FUNCTION "Interfaccia Destacker" : VOID
TITLE =Communication to previous cell
//
VERSION : 0.1

BEGIN
NETWORK
TITLE =Stops Out
//
//
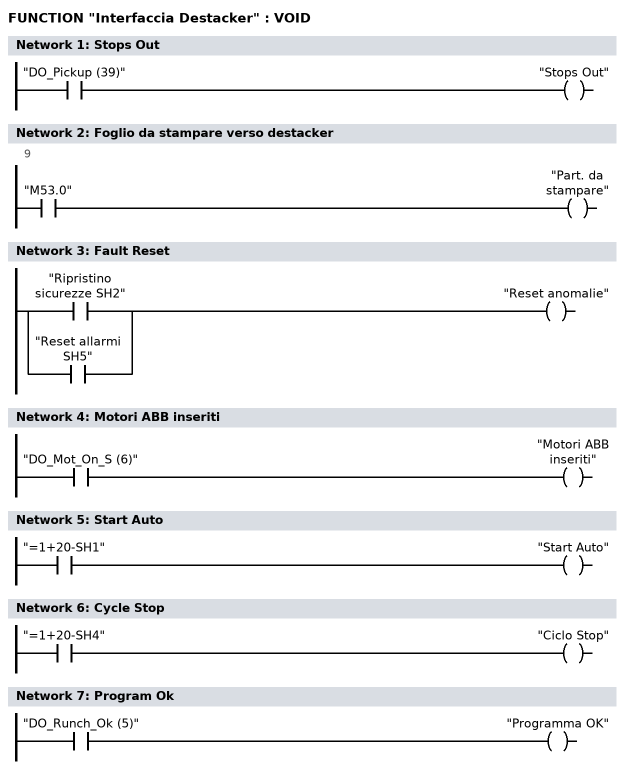
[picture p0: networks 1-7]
      U     "DO_Pickup (39)";
      =     "Stops Out";
NETWORK
TITLE =Foglio da stampare verso destacker
//9
      U     "M53.0";
      =     "Part. da stampare";
NETWORK
TITLE =Fault Reset

      O     "Ripristino sicurezze SH2";
      O     "Reset allarmi SH5";
      =     "Reset anomalie";
NETWORK
TITLE =Motori ABB inseriti

      U     "DO_Mot_On_S (6)";
      =     "Motori ABB inseriti";
NETWORK
TITLE =Start Auto

      U     "=1+20-SH1";
      =     "Start Auto";
NETWORK
TITLE =Cycle Stop

      U     "=1+20-SH4";
      =     "Ciclo Stop";
NETWORK
TITLE =Program Ok

      U     "DO_Runch_Ok (5)";
      =     "Programma OK";
NETWORK
TITLE =Cam Check Double Sheet Sensor

      U(    ;
      U     "vacuostato 1 ok";
      UN    "DO_Pickup (39)";
      L     S5T#1S;
      SE    T      2;
      NOP   0;
      NOP   0;
      NOP   0;
      U     T      2;
      )     ;
      U(    ;
      O     "DO_Motion (40)";
      O     "Selez.ciclo sing.ABB";
      )     ;
      =     "Cam contr. doppio foglio";
NETWORK
TITLE =Mode Selector Programming Mode
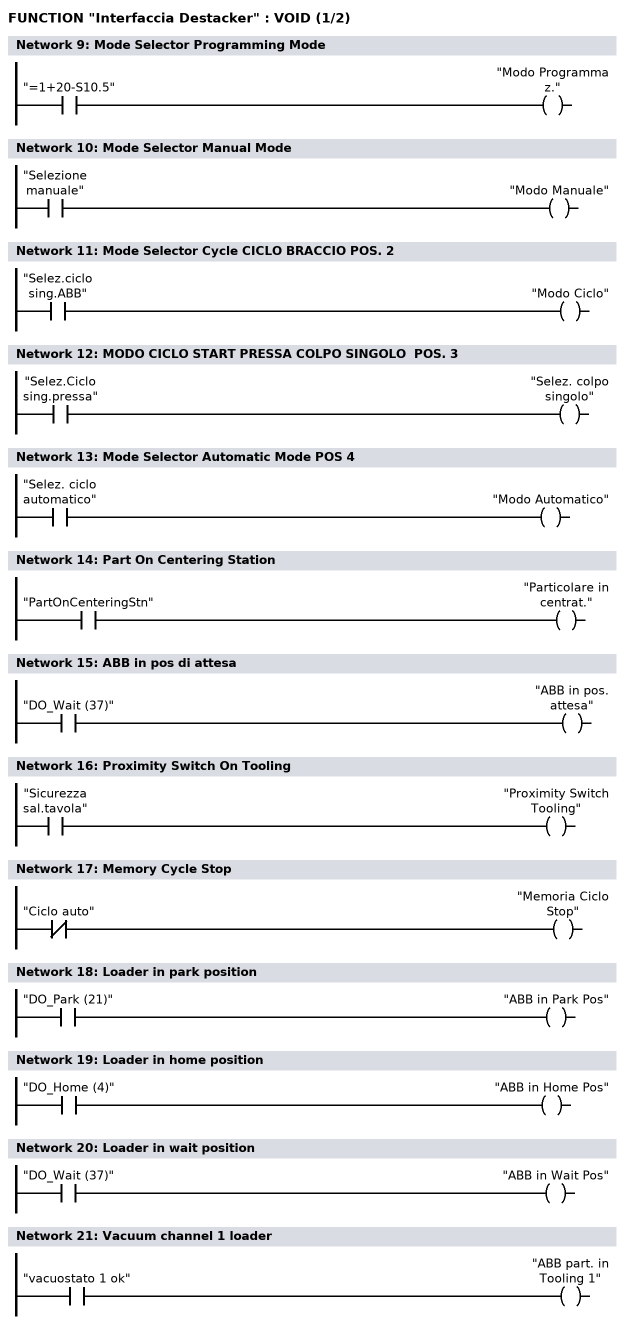
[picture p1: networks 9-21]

      U     "=1+20-S10.5";
      =     "Modo Programmaz.";
NETWORK
TITLE =Mode Selector Manual Mode

      U     "Selezione manuale";
      =     "Modo Manuale";
NETWORK
TITLE =Mode Selector Cycle CICLO BRACCIO POS. 2

      U     "Selez.ciclo sing.ABB";
      =     "Modo Ciclo";
NETWORK
TITLE =MODO CICLO START PRESSA COLPO SINGOLO  POS. 3

      U     "Selez.Ciclo sing.pressa";
      =     "Selez. colpo singolo";
NETWORK
TITLE =Mode Selector Automatic Mode POS 4

      U     "Selez. ciclo automatico";
      =     "Modo Automatico";
NETWORK
TITLE =Part On Centering Station

      U     "PartOnCenteringStn";
      =     "Particolare in centrat.";
NETWORK
TITLE =ABB in pos di attesa

      U     "DO_Wait (37)";
      =     "ABB in pos. attesa";
NETWORK
TITLE =Proximity Switch On Tooling

      U     "Sicurezza sal.tavola";
      =     "Proximity Switch Tooling";
NETWORK
TITLE =Memory Cycle Stop

      UN    "Ciclo auto";
      =     "Memoria Ciclo Stop";
NETWORK
TITLE =Loader in park position

      U     "DO_Park (21)";
      =     "ABB in Park Pos";
NETWORK
TITLE =Loader in home position

      U     "DO_Home (4)";
      =     "ABB in Home Pos";
NETWORK
TITLE =Loader in wait position

      U     "DO_Wait (37)";
      =     "ABB in Wait Pos";
NETWORK
TITLE =Vacuum channel 1 loader

      U     "vacuostato 1 ok";
      =     "ABB part. in Tooling 1";
NETWORK
TITLE =Vacuum channel 2 loader
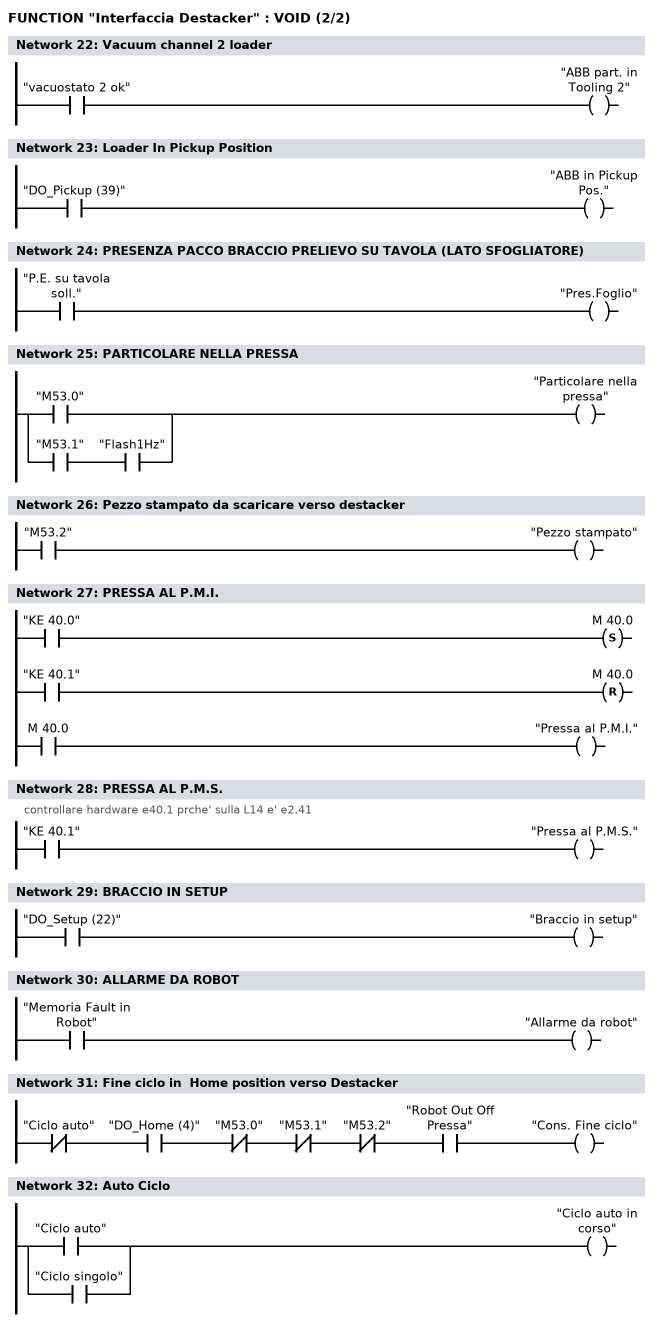
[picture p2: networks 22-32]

      U     "vacuostato 2 ok";
      =     "ABB part. in Tooling 2";
NETWORK
TITLE =Loader In Pickup Position

      U     "DO_Pickup (39)";
      =     "ABB in Pickup Pos.";
NETWORK
TITLE =PRESENZA PACCO BRACCIO PRELIEVO SU TAVOLA (LATO SFOGLIATORE)

      U     "P.E. su tavola soll.";
      =     "Pres.Foglio";
NETWORK
TITLE =PARTICOLARE NELLA PRESSA

      O     "M53.0";
      O     ;
      U     "M53.1";
      U     "Flash1Hz";
      =     "Particolare nella pressa";
NETWORK
TITLE =Pezzo stampato da scaricare verso destacker

      U     "M53.2";
      =     "Pezzo stampato";
NETWORK
TITLE =PRESSA AL P.M.I.

      U     "KE 40.0";
      S     M     40.0;
      U     "KE 40.1";
      R     M     40.0;
      U     M     40.0;
      =     "Pressa al P.M.I.";
NETWORK
TITLE =PRESSA AL P.M.S.
//controllare hardware e40.1 prche' sulla L14 e' e2.41
      U     "KE 40.1";
      =     "Pressa al P.M.S.";
NETWORK
TITLE =BRACCIO IN SETUP

      U     "DO_Setup (22)";
      =     "Braccio in setup";
NETWORK
TITLE =ALLARME DA ROBOT

      U     "Memoria Fault in Robot";
      =     "Allarme da robot";
NETWORK
TITLE =Fine ciclo in  Home position verso Destacker

      UN    "Ciclo auto";
      U     "DO_Home (4)";
      UN    "M53.0";
      UN    "M53.1";
      UN    "M53.2";
      U     "Robot Out Off Pressa";
      =     "Cons. Fine ciclo";
NETWORK
TITLE =Auto Ciclo

      O     "Ciclo auto";
      O     "Ciclo singolo";
      =     "Ciclo auto in corso";
END_FUNCTION

